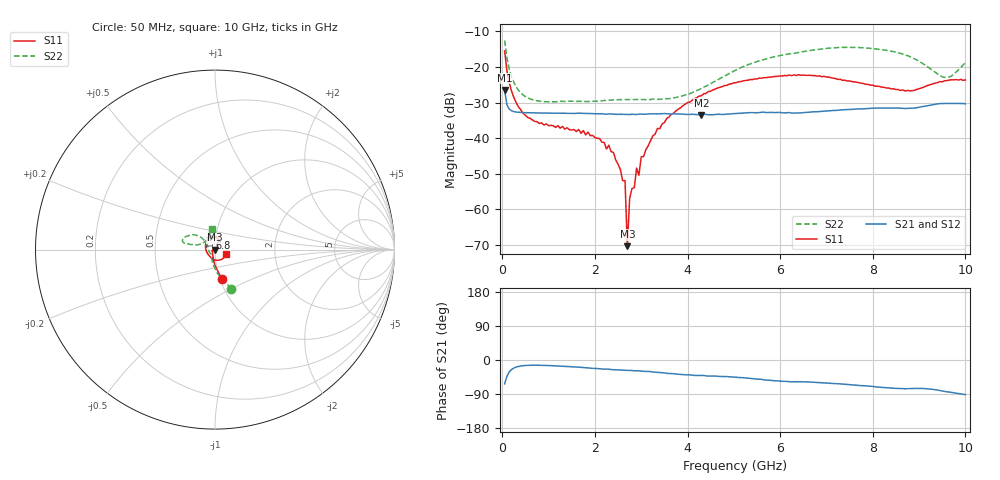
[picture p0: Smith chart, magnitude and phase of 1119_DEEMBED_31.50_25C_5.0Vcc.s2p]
!Hittite Microwave Corp.
!Digital Attenuator/PhaseShifter Rev 1.4.0
!Filename: C:\DATA\DATA\1119_DEEMBED_31.50_25C_5.0Vcc.s2p
!VNA ID: Agilent Technologies,N5224A,MY51441122,A.10.45.03
!Device type:
!2 Port Calibration.
!Temp(C): 25
!Lot Number:
!Serial Number:
!Operator:
!Misc:
!Attenuator:  31.500
# GHZ S DB R 50.0
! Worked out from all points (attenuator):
!   200 points, 50 MHz to 10 GHz, reference 50 ohm
!   highest |S21| = -26.44 dB at 50 MHz (marker M1); lowest = -33.5 dB at 4.3 GHz (marker M2)
!   lowest |S11| = -70.3 dB at 2.7 GHz (marker M3), VSWR 1.00, Z = 50 + j0.0186 ohm
!   |S11| at or under -10 dB: start of sweep to end of sweep
!   |S22| runs from -29.8 to -12.6 dB; largest |S21 - S12| = 0.00011
!   S11 on the Smith chart (normalised r, x): 50 MHz: 1.02, -0.34; 6.8 GHz: 0.93, +0.13; 10 GHz: 1.13, -0.06
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0.05  -15.51 -77.2  -26.44 -63.2  -26.45 -63.2  -12.56 -67.6
0.1  -21.09 -89.9  -30.66 -42.8  -30.67 -42.9  -17.51 -84.0
0.2  -26.77 -103.5  -32.30 -25.1  -32.29 -25.1  -22.77 -100.6
0.45  -33.04 -126.3  -32.82 -15.0  -32.81 -15.1  -27.87 -121.4
0.9  -36.32 -153.5  -32.95 -14.2  -32.95 -14.3  -29.77 -136.0
1.75  -37.86 -167.7  -33.03 -20.0  -33.04 -20.0  -29.68 -141.0
2.3  -41.98 -178.6  -33.19 -24.4  -33.20 -24.6  -29.32 -149.4
2.65  -51.88 139.9  -33.35 -26.9  -33.34 -27.0  -29.14 -154.2
2.7  -70.33 142.3  -33.34 -27.4  -33.34 -27.6  -29.19 -154.6
2.75  -56.94 101.0  -33.36 -27.4  -33.37 -27.5  -29.15 -155.6
2.85  -53.92 54.3  -33.32 -28.5  -33.32 -28.6  -29.17 -158.0
2.9  -48.40 35.7  -33.35 -28.2  -33.36 -28.4  -29.13 -159.2
2.95  -50.44 37.1  -33.25 -28.6  -33.25 -28.7  -29.15 -160.3
3  -45.20 36.4  -33.24 -29.4  -33.26 -29.5  -29.13 -161.8
3.4  -37.34 47.8  -33.16 -32.9  -33.17 -32.9  -29.06 -173.9
4.3  -28.08 56.6  -33.46 -40.6  -33.47 -40.7  -25.99 150.3
5.05  -24.41 69.7  -33.08 -45.4  -33.11 -45.5  -20.84 138.5
6.7  -22.44 111.0  -32.61 -58.6  -32.63 -58.6  -15.27 153.8
6.8  -22.59 113.7  -32.57 -59.4  -32.59 -59.4  -15.12 155.1
8.35  -25.94 -178.1  -31.56 -73.5  -31.57 -73.6  -15.45 168.1
9.55  -23.88 -65.6  -30.25 -82.9  -30.26 -82.9  -22.92 138.1
10  -23.62 -23.0  -30.34 -91.3  -30.35 -91.3  -18.77 98.2
